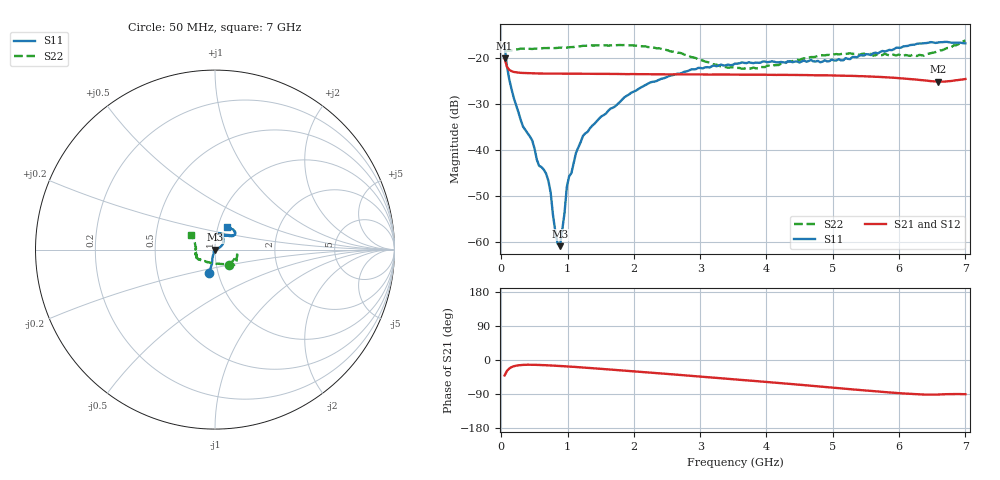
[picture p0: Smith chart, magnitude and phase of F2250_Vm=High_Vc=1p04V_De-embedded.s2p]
! Integrated Device Technology
! Corporate Headquarters
! 6024 Silver Creek Valley Road
! San Jose, CA 95138  USA
! Phone:  1-408-284-8200
! Toll Free:  1-800-223-1366
! Webpage:  http://www.idt.com/
! Timing and RF Division
! 515 Groton Road, Suite 102
! Westford, MA 01886-6024
! Device:  F2250
! Description: Voltage Variable RF Attenuator
! Frequency:  50.0 -  6000.00 MHz
! Package:  3x3 mm Thin QFN Plastic Package: 16 pin
! Ports:  2 RF, 3 DC
!  Pin  1  = GND
!  Pin  2  = NC
!  Pin  3  = RF1  = Port 1
!  Pin  4  = NC
!  Pin  5  = GND
!  Pin  6  = GND
!  Pin  7  = GND
!  Pin  8  = GND
!  Pin  9  = NC
!  Pin 10  = RF2  = Port 2
!  Pin 11  = NC
!  Pin 12  = GND
!  Pin 13  = GND
!  Pin 14  = VCNTRL
!  Pin 15  = VDD
!  Pin 16  = VMODE
! Vcntrl:  1.040 Volts
! Vmode:  +3.300 Volts
! Vdd:  +3.30  Volts
! Current:  1.326 mA
! Data:  The device was measured on a the F2250 evaluation board which has
!  individual transmission lines to the RF pins.  Data was collected
!  using a calibrated network analyzer.  The evaluation board was
!  de-embedded using a TRL calibration technique.
!  The reference plane is the edge of the package pin.
! Misc:  SN 10
!  Action Tracker AT0258
! Date Measured:  2014-11-26
! Date:  2015-10-15  MJV
! Note:
!  Integrated Device Technology supplies this data as a sample of measured
!  data at the package pin for this product.  Your particular data for this
!  product may vary.
!  Data was taken at 25 degrees C.
!  Integrated Device Technology reserves the right to change this data at anytime.
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# GHz S dB R 50
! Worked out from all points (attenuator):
!   201 points, 50 MHz to 7 GHz, reference 50 ohm
!   highest |S21| = -19.99 dB at 50 MHz (marker M1); lowest = -25.1 dB at 6.583 GHz (marker M2)
!   lowest |S11| = -61.0 dB at 884 MHz (marker M3), VSWR 1.00, Z = 50.1 - j0.0564 ohm
!   |S11| at or under -10 dB: start of sweep to end of sweep
!   |S22| runs from -22.3 to -16.1 dB; largest |S21 - S12| = 0.00022
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0.05  -17.33 -104.8  -19.99 -40.9  -19.98 -40.9  -18.81 -47.0
0.1195  -24.56 -104.6  -22.53 -22.5  -22.53 -22.5  -18.31 -17.8
0.29325  -33.46 -109.0  -23.18 -13.3  -23.17 -13.3  -17.90 -13.2
0.467  -37.93 -121.1  -23.27 -12.6  -23.27 -12.6  -17.97 -13.7
0.57125  -43.46 -125.5  -23.32 -13.1  -23.31 -13.0  -17.89 -15.9
0.64075  -44.28 -122.9  -23.33 -13.5  -23.33 -13.5  -17.78 -16.8
0.71025  -46.69 -119.3  -23.34 -14.1  -23.33 -14.1  -17.76 -18.5
0.745  -49.31 -119.1  -23.34 -14.4  -23.34 -14.4  -17.75 -19.1
0.8145  -57.72 -151.7  -23.35 -15.1  -23.35 -15.1  -17.78 -20.8
0.84925  -60.38 -123.9  -23.35 -15.4  -23.34 -15.5  -17.74 -21.8
0.884  -60.95 -39.0  -23.34 -15.8  -23.36 -15.8  -17.71 -22.8
0.9535  -53.74 -49.5  -23.37 -16.5  -23.37 -16.5  -17.73 -23.7
0.98825  -48.06 -24.1  -23.37 -16.9  -23.37 -16.9  -17.68 -24.3
1.12725  -40.59 5.7  -23.38 -18.5  -23.37 -18.5  -17.46 -26.4
1.2315  -36.93 11.0  -23.37 -19.8  -23.36 -19.8  -17.29 -28.5
1.857  -28.49 28.0  -23.43 -28.0  -23.44 -28.0  -17.12 -36.0
2.37825  -24.69 39.2  -23.48 -35.1  -23.47 -35.1  -17.80 -42.4
3.525  -21.16 68.3  -23.57 -51.2  -23.58 -51.2  -22.11 -89.3
4.7065  -20.68 70.3  -23.69 -68.5  -23.69 -68.5  -19.75 -147.3
5.85325  -18.17 38.8  -24.18 -85.6  -24.17 -85.8  -19.35 -169.0
6.583  -16.59 43.5  -25.08 -91.2  -25.07 -91.3  -18.49 160.9
7  -16.75 61.9  -24.52 -90.2  -24.52 -90.3  -16.12 149.4
